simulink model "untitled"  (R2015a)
settings: Solver=ode45  StartTime=0.0  StopTime=5  RelTol=1e-3
libraries: powerlib x7, powerlib_meascontrol x2

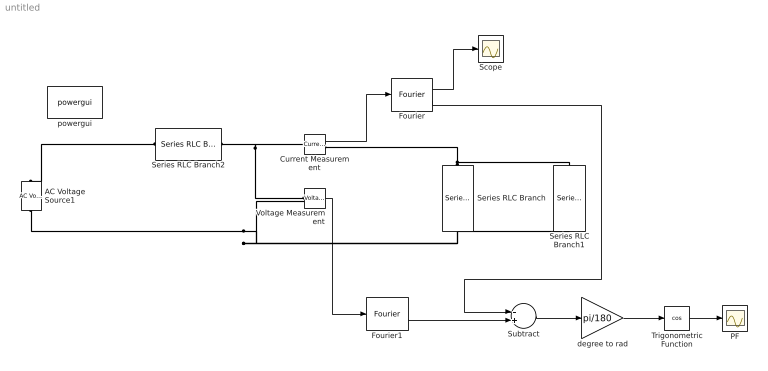
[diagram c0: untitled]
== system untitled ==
  AC Voltage Source1 : powerlib/Electrical Sources/AC Voltage Source  Amplitude=220  Phase=0  Frequency=50  SampleTime=0  Measurements=None
  Current Measurement : powerlib/Measurements/Current Measurement  PhasorSimulation=off  OutputType=Complex  PSBequivalent=0
  Fourier : powerlib_meascontrol/Measurements/Fourier  Freq=60  n=1  InInit=[0, 0]  Ts=0
  Fourier1 : powerlib_meascontrol/Measurements/Fourier  Freq=60  n=1  InInit=[0, 0]  Ts=0
  PF : Scope
  Scope : Scope
  Series RLC Branch : powerlib/Elements/Series RLC Branch  LConnTagsString=__new0  RConnTagsString=__new0  BranchType=RL  Resistance=77  Inductance=250e-3  SetiL0=off  InitialCurrent=0  Capacitance=1e-6  Setx0=off  InitialVoltage=0  Measurements=None
  Series RLC Branch1 : powerlib/Elements/Series RLC Branch  LConnTagsString=__new0  RConnTagsString=__new0  BranchType=C  Resistance=77  Inductance=250e-3  SetiL0=off  InitialCurrent=0  Capacitance=15.6e-6  Setx0=off  InitialVoltage=0  Measurements=None
  Series RLC Branch2 : powerlib/Elements/Series RLC Branch  LConnTagsString=__new0  RConnTagsString=__new0  BranchType=R  Resistance=1  Inductance=490.295e-3  SetiL0=off  InitialCurrent=0  Capacitance=1e-6  Setx0=off  InitialVoltage=0  Measurements=None
  Subtract : Sum  Inputs=-+
  Trigonometric Function : Trigonometry  Operator=cos
  Voltage Measurement : powerlib/Measurements/Voltage Measurement  PhasorSimulation=off  OutputType=Complex  PSBequivalent=0
  degree to rad : Gain  Gain=pi/180
  powergui : powerlib/powergui  Priority=1  SimulationMode=Discrete  SolverType=Tustin/Backward Euler (TBE)  SampleTime=50e-6  frequency=60  SPID=off  DisableSnubberDevices=off  DisableRonSwitches=off  DisableVfSwitches=off  SwTol=0  DisplayEquations=off  Interpol=off  methode=off  Ts=100  FunctionMessages=off  echomessages=off  HookPort=off  EnableUseOfTLC=off  x0status=blocks  frequencyindice=50  Pbase=100e6  ErrMax=1e-4  Iterations=50  UnitsV=kV  UnitsW=MW  buscounter=0  RestoreLinks=warning  ResistiveCurrentMeasurement=off  Frange=[0:2:500]  Ylog=off  Xlog=on  ShowGrid=off  save=off  variable=ZData  structure=0  ZoomFFT=off  StartTime=0.0  cycles=1  DisplayStyle=1  fundamental=60  FreqAxis=off  MaxFrequency=1000  frequencyindicesteady=1  RmsSteady=1  display=off
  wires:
  Current Measurement/1 -> Fourier/1
  Fourier/1 -> Scope/1
  Voltage Measurement/1 -> Fourier1/1
  Fourier1/2 -> Subtract/2
  Fourier/2 -> Subtract/1
  Subtract/1 -> degree to rad/1
  Trigonometric Function/1 -> PF/1
  degree to rad/1 -> Trigonometric Function/1
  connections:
  AC Voltage Source1/LConn1 -- Series RLC Branch1/RConn1 -- Series RLC Branch/RConn1 -- Voltage Measurement/LConn2
  Series RLC Branch/LConn1 -- Series RLC Branch1/LConn1 -- Current Measurement/RConn1
  Voltage Measurement/LConn1 -- Current Measurement/LConn1 -- Series RLC Branch2/RConn1
  Series RLC Branch2/LConn1 -- AC Voltage Source1/RConn1
